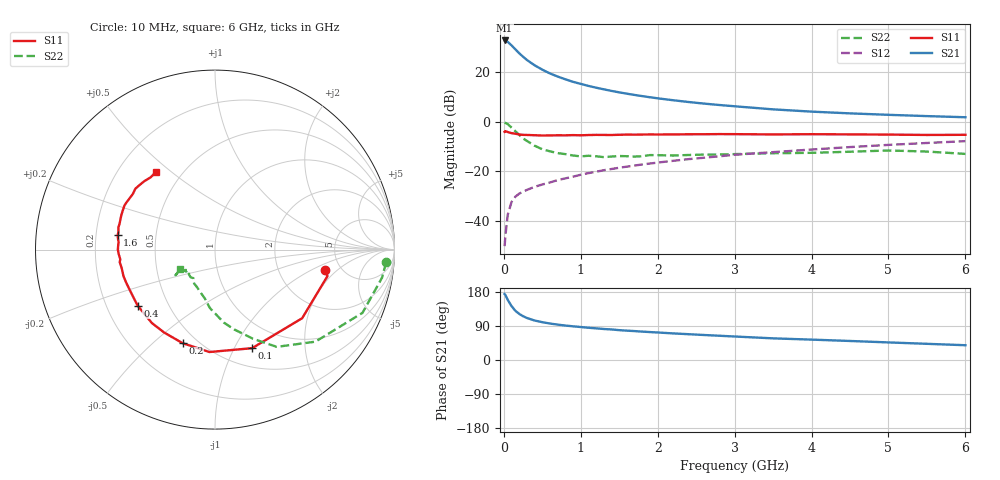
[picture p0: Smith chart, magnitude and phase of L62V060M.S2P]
!  INFINEON TECHNOLOGIES Small Signal Semiconductors
! BFR380L3 , Si-NPN RF-Transistor in TSLP-3-1
!  Vce=2 V,  Ic=60 mA
! Common Emitter S-Parameters:  07. March 2005
#  GHz  S  MA  R  50
! f  S11  S21  S12  S22
! GHz  Mag  Ang  Mag  Ang  Mag  Ang  Mag  Ang
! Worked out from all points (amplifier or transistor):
!   36 points, 10 MHz to 6 GHz, reference 50 ohm
!   highest |S21| = 32.7 dB at 10 MHz (marker M1)
!   |S21| within 3 dB of that: start of sweep to 131.9 MHz
!   unconditionally stable (mu >= 1): 1.381 GHz to 4.902 GHz
!   at 250 MHz: K = 0.50, MSG = 27.2 dB, |S12| = -28.2 dB
!   at 1.4 GHz: K = 1.00, MAG = 15.5 dB, |S12| = -19.1 dB
!   at 6 GHz: K = 0.98, MSG = 4.8 dB, |S12| = -7.9 dB
!   S11 on the Smith chart (normalised r, x): 10 MHz: 3.77, -1.39; 100 MHz: 0.70, -1.18; 200 MHz: 0.42, -0.63; 400 MHz: 0.33, -0.29; 1.6 GHz: 0.29, +0.07; 6 GHz: 0.36, +0.45
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0.01  0.6234 -10.4  43.2 174.0  0.0031 73.9  0.9556 -4.3
0.02  0.6438 -13.3  42.76 171.6  0.005 83.3  0.9439 -9.5
0.05  0.618 -38.2  40.52 158.9  0.0132 75.6  0.8942 -23.2
0.1  0.5868 -69.4  34.41 142.2  0.0241 63.2  0.7592 -42.5
0.15  0.5715 -93.1  28.61 129.9  0.0308 57.0  0.6418 -57.6
0.2  0.5517 -109.1  23.85 121.6  0.0355 54.3  0.5402 -66.9
0.25  0.5419 -121.5  20.3 115.6  0.0387 52.7  0.4581 -76.4
0.3  0.5395 -130.7  17.47 110.9  0.0422 52.3  0.4095 -83.1
0.4  0.5323 -144.1  13.65 104.2  0.0486 53.7  0.3268 -95.0
0.5  0.5256 -152.9  11.15 99.8  0.0542 55.5  0.2783 -101.7
0.6  0.5277 -159.3  9.343 96.2  0.0595 57.3  0.2522 -108.6
0.7  0.5309 -163.8  8.097 93.4  0.0665 59.1  0.2324 -115.4
0.9  0.5354 -172.5  6.34 88.9  0.0779 61.5  0.2079 -126.0
1.1  0.5373 -177.4  5.246 85.1  0.0919 63.6  0.2055 -131.2
1.3  0.5397 177.2  4.477 81.8  0.105 64.6  0.1927 -138.8
1.6  0.5486 171.3  3.653 77.4  0.124 65.3  0.2011 -144.8
2.2  0.5527 162.5  2.701 70.2  0.1625 65.9  0.2078 -146.1
2.8  0.561 154.2  2.164 64.0  0.2004 65.6  0.2176 -151.0
3.5  0.5527 145.9  1.768 57.1  0.243 63.3  0.2312 -149.3
4.5  0.5539 139.9  1.468 50.2  0.3073 61.3  0.2476 -148.1
5.5  0.5393 131.9  1.293 42.7  0.3717 57.3  0.2498 -147.8
6  0.543 126.9  1.226 39.0  0.405 55.0  0.2239 -151.0
